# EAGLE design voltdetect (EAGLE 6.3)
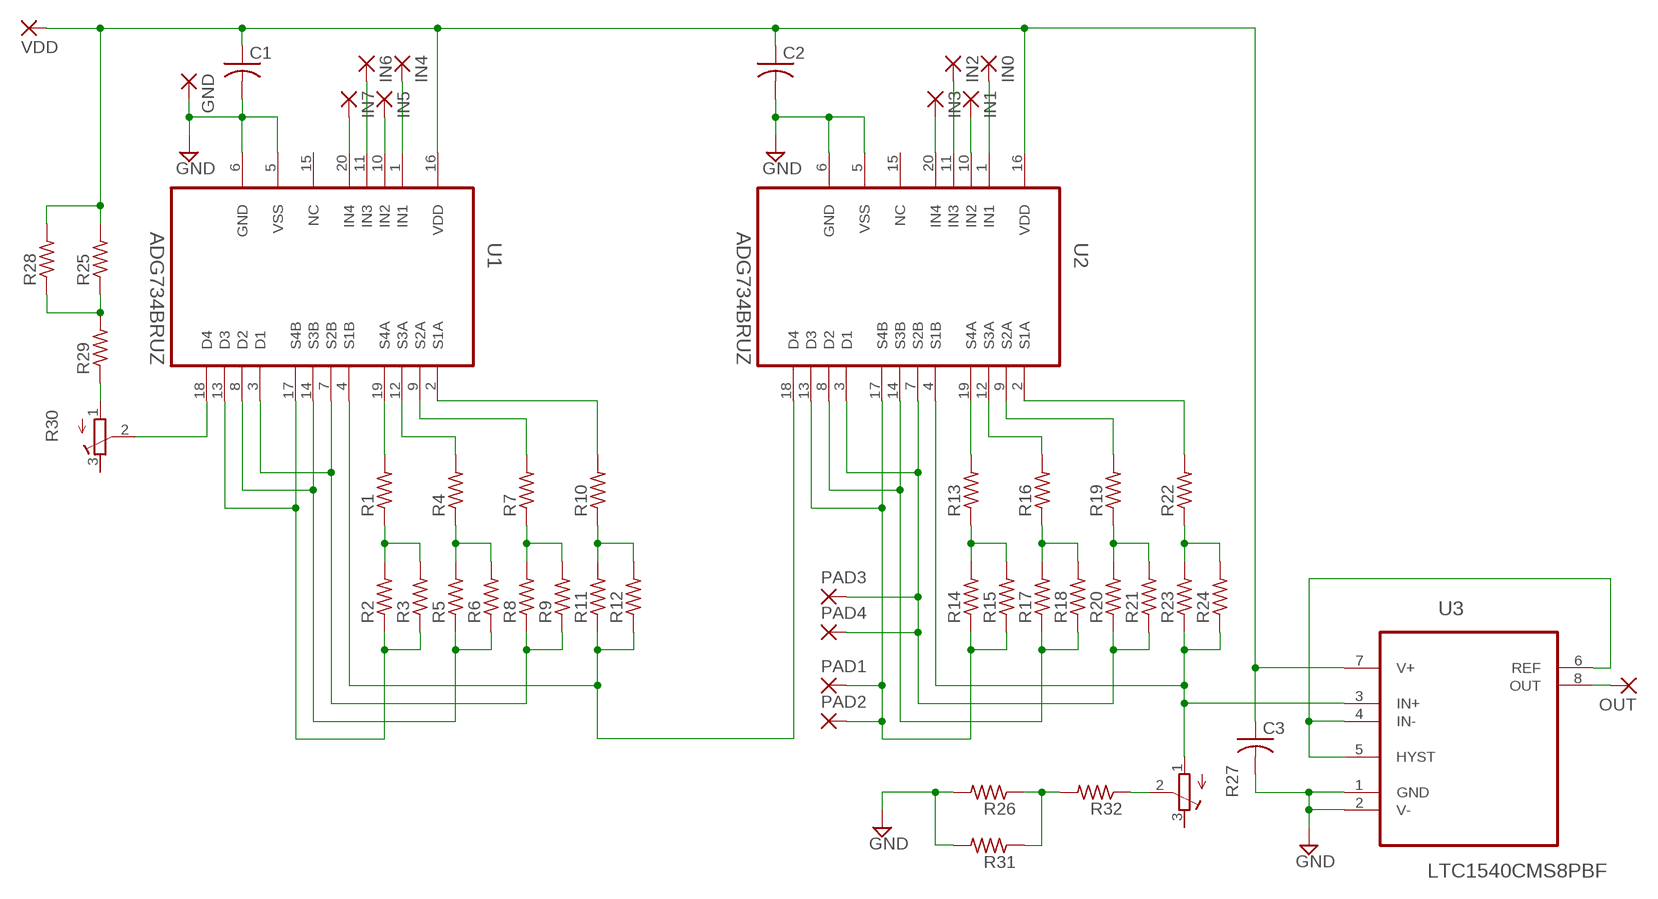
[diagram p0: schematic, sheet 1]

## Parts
C1  C-USC0805  [C0805]
C2  C-USC0805  [C0805]
C3  C-USC0805  [C0805]
GND  SMD5  [SMD2,54-5,08]
IN0  SMD5  [SMD2,54-5,08]
IN1  SMD5  [SMD2,54-5,08]
IN2  SMD5  [SMD2,54-5,08]
IN3  SMD5  [SMD2,54-5,08]
IN4  SMD5  [SMD2,54-5,08]
IN5  SMD5  [SMD2,54-5,08]
IN6  SMD5  [SMD2,54-5,08]
IN7  SMD5  [SMD2,54-5,08]
OUT  SMD5  [SMD2,54-5,08]
PAD1  SMD2  [SMD1,27-2,54]
PAD2  SMD2  [SMD1,27-2,54]
PAD3  SMD2  [SMD1,27-2,54]
PAD4  SMD2  [SMD1,27-2,54]
R1  R-US_M0805  [M0805]
R2  R-US_M0805  [M0805]
R3  R-US_M0805  [M0805]
R4  R-US_M0805  [M0805]
R5  R-US_M0805  [M0805]
R6  R-US_M0805  [M0805]
R7  R-US_M0805  [M0805]
R8  R-US_M0805  [M0805]
R9  R-US_M0805  [M0805]
R10  R-US_M0805  [M0805]
R11  R-US_M0805  [M0805]
R12  R-US_M0805  [M0805]
R13  R-US_M0805  [M0805]
R14  R-US_M0805  [M0805]
R15  R-US_M0805  [M0805]
R16  R-US_M0805  [M0805]
R17  R-US_M0805  [M0805]
R18  R-US_M0805  [M0805]
R19  R-US_M0805  [M0805]
R20  R-US_M0805  [M0805]
R21  R-US_M0805  [M0805]
R22  R-US_M0805  [M0805]
R23  R-US_M0805  [M0805]
R24  R-US_M0805  [M0805]
R25  R-US_M0805  [M0805]
R26  R-US_M0805  [M0805]
R27  R-TRIMM3224J  [RTRIM3224J]
R28  R-US_M0805  [M0805]
R29  R-US_M0805  [M0805]
R30  R-TRIMM3224J  [RTRIM3224J]
R31  R-US_M0805  [M0805]
R32  R-US_M0805  [M0805]
U1  ADG734BRUZ  [SOP65P640X120-20N]
U2  ADG734BRUZ  [SOP65P640X120-20N]
U3  LTC1540CMS8PBF  [SOP65P490X110-8N]
VDD  SMD5  [SMD2,54-5,08]

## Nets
GND: C1.2 C2.2 C3.2 GND.1(P) R26.2 R31.2 U1.5(VSS) U1.6(GND) U2.5(VSS) U2.6(GND) U3.1(GND) U3.2(V-)
N$1: R1.1 R2.2 R3.2
N$2: R13.1 R14.2 R15.2
N$3: R4.1 R5.2 R6.2
N$4: R16.1 R17.2 R18.2
N$5: R7.1 R8.2 R9.2
N$6: R19.1 R20.2 R21.2
N$7: R10.1 R11.2 R12.2
N$8: R22.1 R23.2 R24.2
N$9: PAD1.1(P) PAD2.1(P) R14.1 R15.1 U2.13(D3) U2.17(S4B)
N$10: R17.1 R18.1 U2.8(D2) U2.14(S3B)
N$11: PAD3.1(P) PAD4.1(P) R20.1 R21.1 U2.3(D1) U2.7(S2B)
N$12: R2.1 R3.1 U1.13(D3) U1.17(S4B)
N$13: R5.1 R6.1 U1.8(D2) U1.14(S3B)
N$14: R8.1 R9.1 U1.3(D1) U1.7(S2B)
N$15: R11.1 R12.1 U1.4(S1B) U2.18(D4)
N$16: R23.1 R24.1 R27.1(A) U2.4(S1B) U3.3(IN+)
N$17: R13.2 U2.19(S4A)
N$18: R16.2 U2.12(S3A)
N$19: R19.2 U2.9(S2A)
N$20: R1.2 U1.19(S4A)
N$21: R4.2 U1.12(S3A)
N$22: R7.2 U1.9(S2A)
N$23: R10.2 U1.2(S1A)
N$24: R30.2(S) U1.18(D4)
N$25: R22.2 U2.2(S1A)
N$26: IN3.1(P) U2.20(IN4)
N$27: IN2.1(P) U2.11(IN3)
N$28: IN1.1(P) U2.10(IN2)
N$29: IN0.1(P) U2.1(IN1)
N$30: IN7.1(P) U1.20(IN4)
N$31: IN6.1(P) U1.11(IN3)
N$32: IN5.1(P) U1.10(IN2)
N$33: IN4.1(P) U1.1(IN1)
N$34: R25.1 R28.1 R29.2
N$35: R26.1 R31.1 R32.2
N$36: R27.2(S) R32.1
N$37: U3.4(IN-) U3.5(HYST) U3.6(REF)
N$38: C1.1 C2.1 C3.1 R25.2 R28.2 U1.16(VDD) U2.16(VDD) U3.7(V+) VDD.1(P)
N$40: R29.1 R30.1(A)
OUT: OUT.1(P) U3.8(OUT)
Unconnected: R27.3(E) R30.3(E) U1.15(NC) U2.15(NC)

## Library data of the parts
C1-C3 = rcl:C-US: CAPACITOR, American symbol
GND IN0 IN1-IN7 OUT VDD = wirepad:SMD5: SMD PAD
PAD1-PAD4 = wirepad:SMD2: SMD PAD
R1-R26 R28 R29 R31 R32 = rcl:R-US_: RESISTOR, American symbol
R27 R30 = rcl:R-TRIMM: Trimm resistor
U1 U2 = Analog Devices_By_element14_Batch_1:ADG734BRUZ: CMOS, 2.5Low Voltage, Triple/Quad SPDT Switches; MPN: ADG734BRUZ; OC_FARNELL: 1661037; OC_NEWARK: 59K1572; PACKAGE: TSSOP-20; SUPPLIER: Analog devices
U3 = LTC_By_element14_Batch_1:LTC1540CMS8PBF: Nanopower Comparator with Reference; MPN: LTC1540CMS8#PBF; OC_FARNELL: 1663643; OC_NEWARK: 56M1861; PACKAGE: MSOP-8; SUPPLIER: Linear Technology

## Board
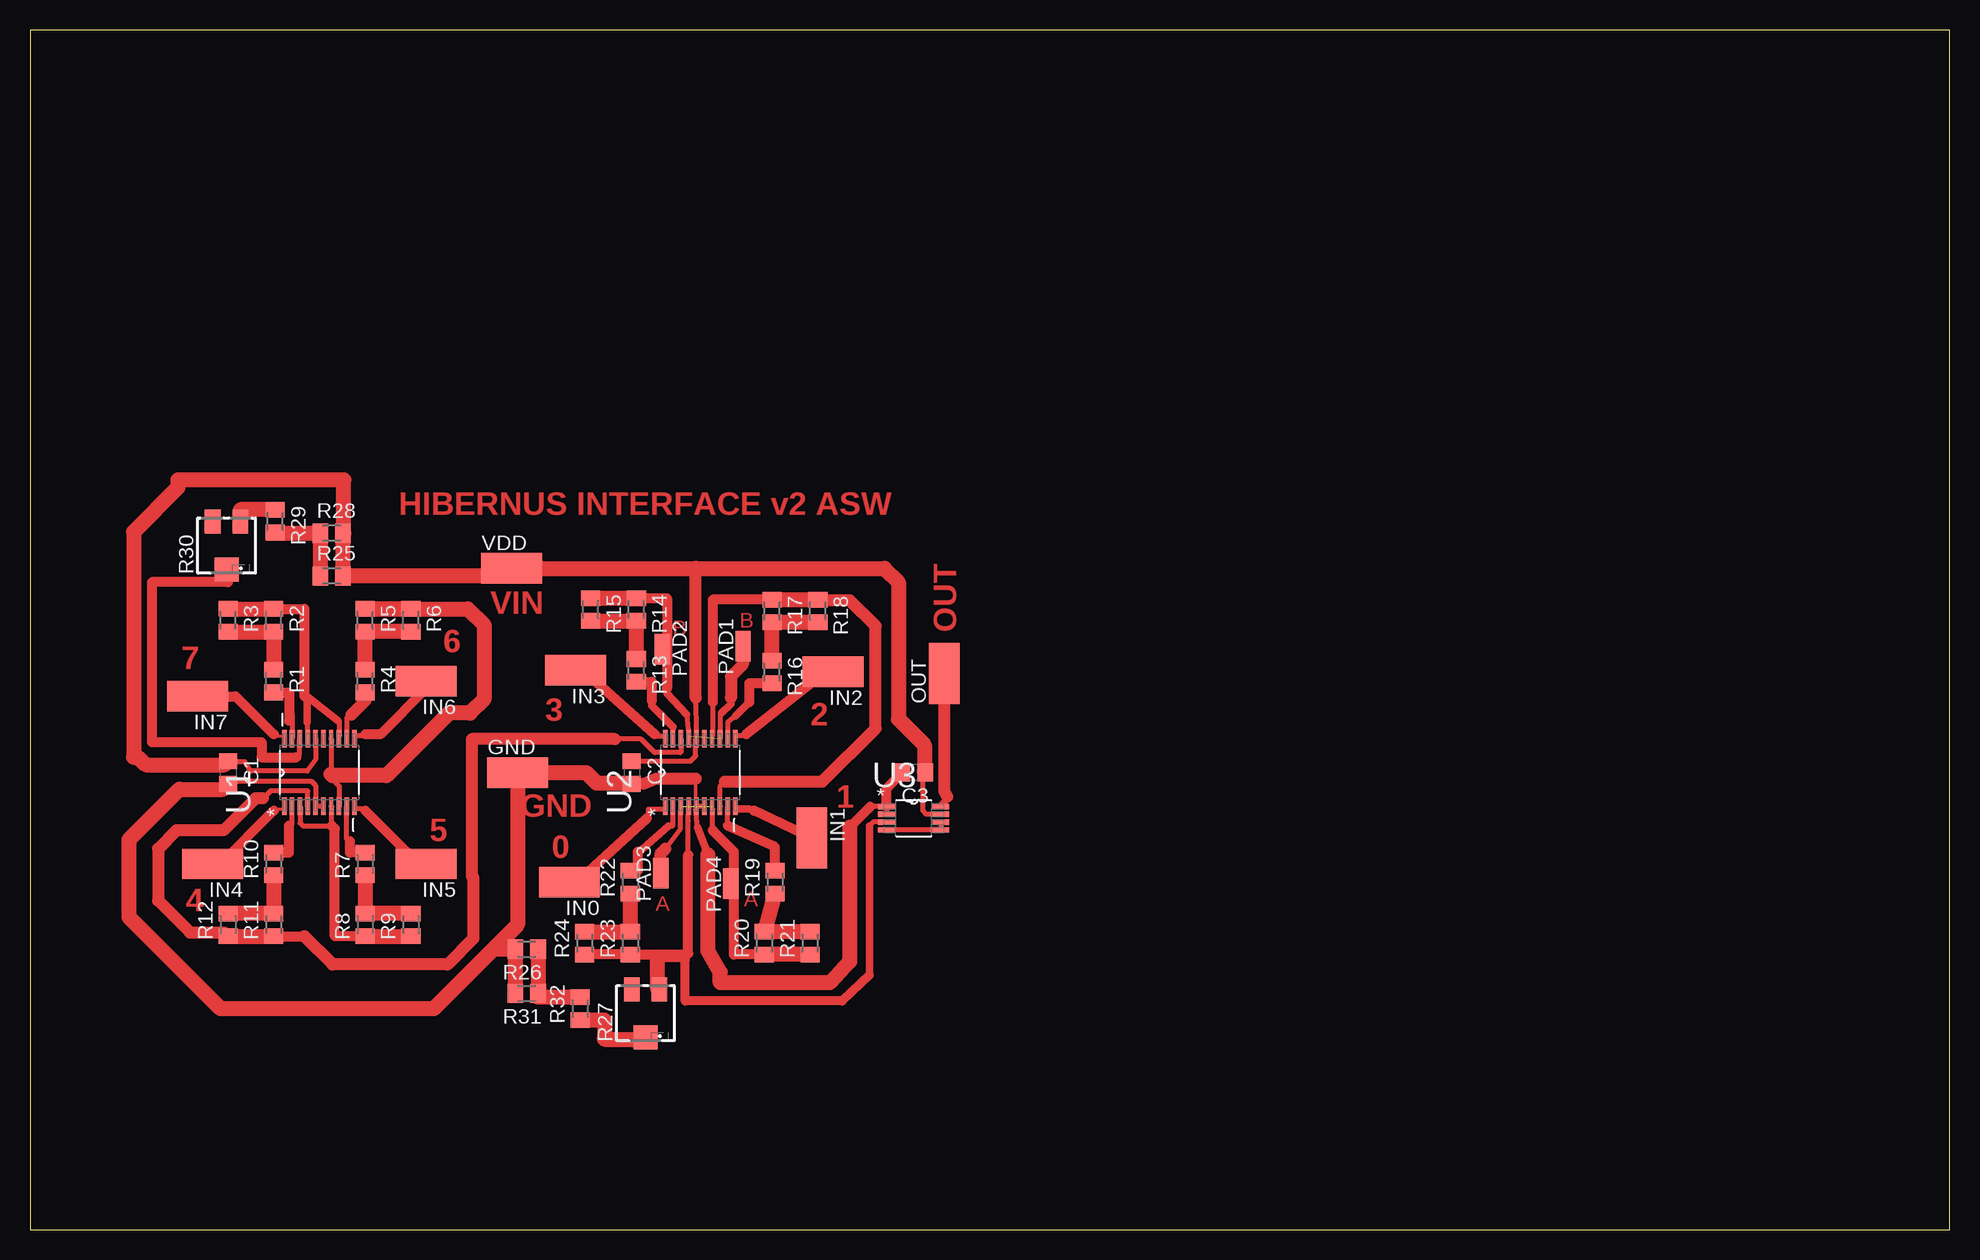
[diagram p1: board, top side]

Size 160 x 100 mm. Coordinates in mm from the lower left corner, seen from the top.
Outline: 0,0 160,0 160,100 0,100 0,0
Copper layers (1*16): Top 0.035mm / dielectric 1.5mm / Bottom 0.035mm
Design rules "default": minimum track width 10mil, minimum drill 24mil, track to track 8mil, track to pad 8mil, pad to pad 8mil, via to via 8mil, smd to smd 8mil, copper to edge 40mil, drill to drill 8mil, minimum pad ring 10mil, minimum via ring 8mil, stop-mask expansion 4mil, vias tented up to drill 0mil, thermal gap 10mil

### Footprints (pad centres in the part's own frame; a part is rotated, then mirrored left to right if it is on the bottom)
C0805 = smd 1.3 x 1.5: 1 -0.95,0; 2 0.95,0
SMD2,54-5,08 = smd 2.54 x 5.08: 1 0,0
SMD1,27-2,54 = smd 1.27 x 2.54: 1 0,0
M0805 = smd 1.3 x 1.6: 1 -0.95,0; 2 0.95,0
RTRIM3224J = smd 1.3 x 2: 1 -1.15,-2; 3 1.15,-2 | smd 2 x 2: 2 0,2
SOP65P640X120-20N = smd 1.473 x 0.356: 1 -2.819,2.921; 2 -2.819,2.286; 3 -2.819,1.626; 4 -2.819,0.965; 5 -2.819,0.33; 6 -2.819,-0.33; 7 -2.819,-0.965; 8 -2.819,-1.626; 9 -2.819,-2.286; 10 -2.819,-2.921; 11 2.819,-2.921; 12 2.819,-2.286; 13 2.819,-1.626; 14 2.819,-0.965; 15 2.819,-0.33; 16 2.819,0.33; 17 2.819,0.965; 18 2.819,1.626; 19 2.819,2.286; 20 2.819,2.921
SOP65P490X110-8N = smd 1.397 x 0.432: 1 -2.261,0.965; 2 -2.261,0.33; 3 -2.261,-0.33; 4 -2.261,-0.965; 5 2.261,-0.965; 6 2.261,-0.33; 7 2.261,0.33; 8 2.261,0.965

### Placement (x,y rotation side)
C1  16.51,38.1 270 top
C2  50.16,38.1 270 top
C3  73.66,38.1 180 top
GND  40.64,38.1 270 top
IN0  44.96,28.96 90 top
IN1  65.15,32.64 180 top
IN2  66.93,46.48 90 top
IN3  45.47,46.61 90 top
IN4  15.24,30.48 90 top
IN5  33.02,30.48 90 top
IN6  33.02,45.72 90 top
IN7  13.97,44.45 90 top
OUT  76.2,46.35 0 top
PAD1  59.44,48.64 0 top
PAD2  52.7,48.39 180 top
PAD3  52.58,29.72 0 top
PAD4  58.42,28.83 0 top
R1  20.32,45.72 270 top
R2  20.32,50.8 270 top
R3  16.51,50.8 270 top
R4  27.94,45.72 270 top
R5  27.94,50.8 270 top
R6  31.75,50.8 270 top
R7  27.94,30.48 90 top
R8  27.94,25.4 90 top
R9  31.75,25.4 90 top
R10  20.32,30.48 90 top
R11  20.32,25.4 90 top
R12  16.51,25.4 90 top
R13  50.55,46.61 270 top
R14  50.55,51.69 270 top
R15  46.74,51.69 270 top
R16  61.85,46.48 270 top
R17  61.85,51.56 270 top
R18  65.66,51.56 270 top
R19  62.1,28.96 90 top
R20  61.21,23.88 90 top
R21  65.02,23.88 90 top
R22  50.04,28.96 90 top
R23  50.04,23.88 90 top
R24  46.23,23.88 90 top
R25  25.15,54.48 0 top
R26  41.4,23.37 180 top
R27  51.31,18.03 180 top
R28  25.15,58.04 0 top
R29  20.45,59.05 270 top
R30  16.38,57.02 180 top
R31  41.4,19.68 180 top
R32  45.85,18.41 90 top
U1  24.13,38.1 90 top
U2  55.88,38.1 90 top
U3  73.66,34.29 0 top
VDD  40.13,55.12 270 top

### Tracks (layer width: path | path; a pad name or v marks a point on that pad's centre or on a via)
GND
  Top 0.254: 56.13,35.31 U2.6 | 55.63,35.31 U2.5 55.5,35.05
  Top 0.305: 55.5,37.59 55.5,35.33
  Top 0.406: C2.2 51.12,37.15 | 55.5,35.33 U2.5 | C1.2 16.7,37.34 23.5,37.34 23.8,37.03 U1.5 U1.6 | U3.2 U3.1 70.05,35.26 | 55.63,35.31 56.13,35.31 | 55.63,33.53 55.5,35.05
  Top 0.61: 55.63,33.53 56.52,31.24
  Top 0.813: U3.1 71.4,36.79 C3.2 | 70.05,35.26 68.33,33.53
  Top 1.016: 51.12,37.15 52.2,37.59 55.5,37.59
  Top 1.27: C2.2 50.1,37.21 47.24,37.21 46.35,38.1 GND.1 40.64,25.4 38.61,23.37 | C1.2 16.06,36.7 12.45,36.7 8.26,32.51 8.26,26.04 15.88,18.41 33.66,18.41 38.23,22.99 38.61,23.37 | 68.33,33.53 68.33,22.35 66.67,20.57 57.53,20.57 57.53,21.46 56.52,23.24 56.52,31.24 | 38.61,23.37 R26.2 R31.2
N$1
  Top 0.254: 16.51,49.78 R3.2 | 19.81,49.78 R2.2
  Top 1.27: R2.2 R1.1 | 19.81,49.78 16.51,49.78
N$2
  Top 1.27: R15.2 R14.2 R13.1
N$3
  Top 1.27: R6.2 R5.2 R4.1
N$4
  Top 1.27: R16.1 R17.2 R18.2
N$5
  Top 1.27: R7.1 R8.2 R9.2
N$6
  Top 1.27: R19.1 R20.2 R21.2
N$7
  Top 1.27: R10.1 R11.2 R12.2
N$8
  Top 1.27: R22.1 R23.2 R24.2
N$9  (1 unrouted)
  Top 0.254: 54.86,41.66 54.99,41.15 54.86,41.15 U2.17 | 53.09,44.7 53.09,45.09
  Top 0.406: 54.74,42.93 54.86,41.66 | 58.42,44.32 58.42,43.81 | 57.66,43.05 57.53,43.05 57.53,40.95 U2.13 | PAD2.1 53.21,45.47 53.09,45.34
  Top 0.61: 53.09,44.7 54.74,42.93 | 58.42,43.81 57.66,43.05
  Top 0.813: R14.1 53.09,52.64 53.09,45.34 53.09,45.09
  Top 1.016: PAD1.1 59.44,47.12 58.42,46.1 58.42,44.32
  Top 1.27: R15.1 R14.1
N$10
  Top 0.254: 56.9,41.15 U2.14
  Top 0.406: U2.8 57.53,35.31 57.53,36.96 57.91,37.34 | 56.9,43.94 56.9,41.15
  Top 0.813: R17.1 56.9,52.51 56.9,43.94
  Top 1.016: 57.91,37.34 66.04,37.34 70.48,41.78 70.48,50.29 68.33,52.45 65.72,52.45 R18.1
  Top 1.27: R17.1 R18.1
N$11  (1 unrouted)
  Top 0.254: 56.9,35.05 U2.7 | PAD4.1 58.42,28.96 58.67,28.96
  Top 0.406: 56.9,33.27 56.9,35.05 | 52.96,31.75 54.23,33.4 54.23,34.62 U2.3
  Top 0.813: R20.1 58.67,22.93 58.67,28.96 58.67,31.5 56.9,33.27
  Top 1.016: PAD3.1 52.58,31.37 52.96,31.75
  Top 1.27: R21.1 R20.1
N$12
  Top 0.254: 23.11,44.2 22.86,44.45 23.11,44.45 | 25.78,41.15 U1.13
  Top 0.406: 23.11,42.29 U1.17 | 25.65,42.42 25.78,42.42 25.78,41.15
  Top 0.61: 23.11,44.2 23.11,42.29 | 23.11,44.45 25.65,42.42
  Top 0.813: R2.1 22.86,51.75 22.86,44.45
  Top 1.27: R3.1 R2.1
N$13
  Top 0.406: U1.14 25.09,37.97 25.09,37.64 25.78,36.96 25.78,35.31 U1.8
  Top 1.27: R6.1 R5.1 36.52,51.75 37.85,50.42 37.85,44.2 36.7,43.05 34.92,43.05 29.72,37.85 25.22,37.85 25.09,37.97
N$14
  Top 0.406: U1.3 22.5,33.88 22.73,33.66 25.15,33.66 25.15,35.23 U1.7
  Top 0.813: R8.1 25.4,24.45 25.4,33.4 25.15,33.66
  Top 1.27: R8.1 R9.1
N$15
  Top 0.406: U2.18 54.25,39.78 54.23,39.75 52.07,39.75 50.93,40.89 48.77,40.89 | U1.4 23.16,36.52 23.11,36.58 20.07,36.58 19.43,35.94
  Top 0.813: R11.1 22.86,24.45
  Top 1.016: 48.77,40.89 36.83,40.89 36.83,29.46 36.96,29.34 36.96,24.26 34.8,22.1 25.21,22.1 22.86,24.45 | 19.43,35.94 18.8,35.94 16.13,33.27 12.19,33.27 10.67,31.75 10.67,27.43 13.34,24.77 16.2,24.77 R12.1
  Top 1.27: R12.1 R11.1
N$16
  Top 0.406: U3.3 70.28,33.96 69.98,33.66 | 54.61,22.48 52.32,22.48 52.07,22.48 54.86,22.99 | 54.86,31.24 54.86,34.04 U2.4
  Top 0.61: 69.98,33.66 69.98,21.21
  Top 0.762: 69.98,21.21 67.69,19.05 54.61,19.05 54.61,22.48
  Top 0.813: 54.86,31.24 54.86,22.99 51.94,22.93 R23.1 R24.1 46.21,22.93
  Top 1.27: R27.1 52.32,20.03 52.32,22.48
N$17
  Top 0.254: 53.59,41.91 U2.19 | 51.82,43.69 51.82,44.07
  Top 0.61: 51.82,43.69 53.59,41.91
  Top 0.813: R13.2 51.82,45.66 51.82,44.07
N$18
  Top 0.406: 58.8,42.8 58.17,42.29 U2.12
  Top 0.61: 59.94,43.94 58.8,42.8
  Top 0.813: R16.2 59.94,45.53 59.94,43.94
N$19
  Top 0.406: 58.17,33.66 U2.9
  Top 0.813: R19.2 62.1,31.88 58.17,33.66
N$20
  Top 0.254: 21.84,42.93 21.59,42.42
  Top 0.406: 21.84,42.93 U1.19
  Top 0.813: R1.2 21.59,44.77 21.59,42.42
N$21
  Top 0.254: 26.42,42.67 26.8,42.93
  Top 0.406: 26.42,42.67 U1.12
  Top 1.016: R4.2 27.94,44.07 26.8,42.93
N$22
  Top 0.254: 26.42,32.51 26.67,32.38
  Top 0.406: 26.42,32.51 U1.9
  Top 0.813: R7.2 26.67,31.43 26.67,32.38
N$23
  Top 0.254: 21.84,33.78 21.59,33.66
  Top 0.406: 21.84,33.78 U1.2
  Top 0.813: R10.2 21.59,31.43 21.59,33.66
N$24
  Top 0.254: 22.48,40.89 U1.18 | 22.48,39.62 22.23,39.37 | 16.51,53.98 16.51,54.86 R30.2
  Top 0.406: 22.48,39.62 22.48,40.89
  Top 0.813: 16.51,53.98 10.16,53.98 10.16,40.64 19.3,40.64 19.3,39.37 22.23,39.37
N$25
  Top 0.254: 51.05,31.75 51.05,31.5 50.67,31.5
  Top 0.406: 53.21,33.66 53.59,33.66 U2.2
  Top 0.61: 51.05,31.75 53.21,33.66
  Top 0.813: R22.2 50.67,29.91 50.67,31.5
N$26
  Top 0.254: 52.83,41.15 U2.20 | 52.32,41.15 52.07,41.27
  Top 0.406: 52.32,41.15 52.83,41.15
  Top 0.813: IN3.1 46.1,46.61 52.07,41.27
N$27
  Top 0.254: 58.93,41.15 U2.11 | 59.44,41.15 59.69,41.27
  Top 0.406: 59.44,41.15 58.93,41.15
  Top 0.813: IN2.1 66.29,46.48 59.69,41.27
N$28
  Top 0.254: 58.93,35.05 U2.10 | 59.94,35.05 60.33,34.92
  Top 0.61: 59.94,35.05 58.93,35.05
  Top 0.813: IN1.1 60.33,34.92
N$29
  Top 0.254: 52.83,35.05 U2.1 | 51.56,34.54 51.44,34.29
  Top 0.406: 52.83,35.05 51.56,35.05 51.56,34.54
  Top 0.813: IN0.1 45.59,28.96 51.44,34.29
N$30
  Top 0.254: U1.20 21.08,41.15 20.57,41.15 20.32,41.27
  Top 0.813: IN7.1 17.14,44.45 20.32,41.27
N$31
  Top 0.254: 27.18,41.15 U1.11 | 27.69,41.15 27.94,41.27
  Top 0.406: 27.69,41.15 27.18,41.15
  Top 0.813: IN6.1 33.02,45.09 29.21,41.27 27.94,41.27
N$32
  Top 0.254: 27.18,35.05 U1.10 | 27.69,35.05 27.94,34.92
  Top 0.406: 27.69,35.05 27.18,35.05
  Top 0.813: IN5.1 32.38,30.48 27.94,34.92
N$33
  Top 0.254: U1.1 21.08,35.05 20.57,35.05 20.32,34.92
  Top 0.813: IN4.1 15.88,30.48 20.32,34.92
N$34
  Top 1.27: R25.1 R28.1 20.45,58.04 R29.2
N$35
  Top 1.27: R26.1 R31.1 42.35,19.36 R32.2
N$36
  Top 1.27: R32.1 47.88,17.46 47.88,15.88 51.31,15.88 R27.2
N$37
  Top 0.406: U3.6 U3.5 U3.4
N$38
  Top 0.254: C3.1 74.68,38.1 74.55,38.16
  Top 0.406: U3.7 74.73,34.62 74.42,34.92 74.42,37.91 C3.1 | 72.39,42.55 72.26,42.67 | C2.1 55.05,39.05 55.5,39.5 55.5,40.87 U2.16 55.55,42.34 55.5,44.32 | U1.16 23.8,39.17 23.11,38.23 18.41,38.23 17.91,38.99 16.57,38.99 C1.1
  Top 1.016: 55.5,44.32 55.5,55.12
  Top 1.27: 74.55,38.16 74.55,40.39 72.39,42.55 72.39,53.98 71.25,55.12 55.5,55.12 VDD.1 39.37,54.48 R25.2 R28.2 26.16,58.04 26.16,62.48 12.32,62.48 12.32,61.85 8.64,58.17 8.64,39.37 9.02,39.37 9.65,38.73 16.2,38.73 C1.1
N$40
  Top 1.27: R29.1 17.53,60.01 R30.1
OUT
  Top 0.254: 76.2,35.56 76.2,35.81 76.45,36.07 | 75.95,35.31 U3.8
  Top 0.61: 76.2,35.56 75.95,35.31
  Top 1.016: OUT.1 76.2,36.58 76.45,36.07

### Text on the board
Top: HIBERNUS INTERFACE v2 ASW | VIN | B | B | 6 | OUT | 7 | 3 | 2 | 1 | GND | 5 | 0 | 4 | A | A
